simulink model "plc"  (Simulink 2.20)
settings: Solver=ode45  StartTime=0.0  StopTime=1000  RelTol=1e-3  AbsTol=1e-6
undefined symbols (not defined in the file or in its folder): Manual

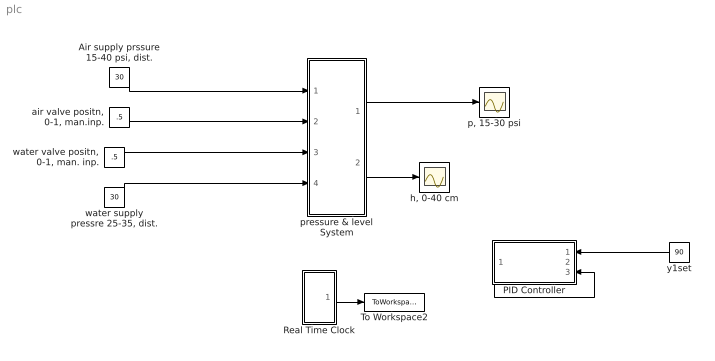
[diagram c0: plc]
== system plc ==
  "Air supply prssure 15-40 psi, dist." : Constant  Value=30
  PID Controller : Subsystem  Orientation=left  mask(Real PID Controller){am_flag=Manual, co=1, Ts=1, Kc=1, taui=10000, taud=0, co_max=100, co_min=0, al=0}
      mask prompts: am_flag "Auto/Manual Switch"; co "Manual Controller Output"; Ts "Sample Time,Ts"; Kc "Kc: Proportional Gain: Negative for DIRECT Action"; taui "taui: Integral time"; taud "Derivative Time, taud"; co_max "Upper limit for controller output"; co_min "Lower limit for controller output"; al "Noise filter tim const, al"
      mask help: Programmed by Babu Joseph, Washington Universtiy in St. Louis, 1998
  Real Time Clock : Subsystem  mask(Sample time){Ts=1}
      mask prompts: Ts "Sample time"
      mask help: This block is used to set the sample time.
  To Workspace2 : ToWorkspace  VariableName=t  SampleTime=1
  "air valve positn, 0-1, man.inp." : Constant  Value=.5
  "h, 0-40 cm" : Scope
  "p, 15-30 psi" : Scope
  pressure & level System : Subsystem  mask{A=100, hinit=20, pinit=25, Ts=1}
      mask prompts: A "area"
  "water supply pressre 25-35, dist." : Constant  Value=30
  "water valve positn, 0-1, man. inp." : Constant  Value=.5
  y1set : Constant  Orientation=left  Value=90
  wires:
  "Air supply prssure 15-40 psi, dist."/1 -> pressure & level System/1(In1)
  pressure & level System/1(p) -> "p, 15-30 psi"/1
  "air valve positn, 0-1, man.inp."/1 -> pressure & level System/2(In2)
  y1set/1 -> PID Controller/1(setpt)
  ? -> PID Controller/2(meas)
  PID Controller/1(output) -> PID Controller/3(out_fdbk)
  Real Time Clock/1("Clock ") -> To Workspace2/1
  "water valve positn, 0-1, man. inp."/1 -> pressure & level System/3(xw)
  "water supply pressre 25-35, dist."/1 -> pressure & level System/4(pw)
  pressure & level System/2(h) -> "h, 0-40 cm"/1

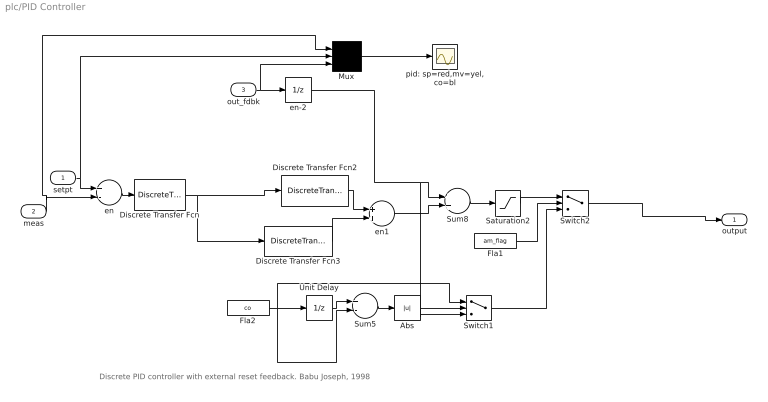
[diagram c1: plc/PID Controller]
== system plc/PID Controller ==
  note: Discrete PID controller with external reset feedback. Babu Joseph, 1998
  setpt : Inport  Port=1  PortWidth=-1  SampleTime=-1
  meas : Inport  Port=2  PortWidth=-1  SampleTime=-1
  out_fdbk : Inport  Port=3  PortWidth=-1  SampleTime=-1
  Abs : Abs
  Discrete Transfer Fcn : DiscreteTransferFcn  Numerator="[Ts   0]"  Denominator="[(al+Ts)  -al]"  SampleTime=Ts
  Discrete Transfer Fcn2 : DiscreteTransferFcn  Numerator="Kc*[ (1+Ts/taui)  -1 ]"  Denominator="[ 1  0 ]"  SampleTime=Ts
  Discrete Transfer Fcn3 : DiscreteTransferFcn  Numerator=Kc*taud*[1 -2 1]  Denominator=[ 1 0 0]  SampleTime=Ts
  Fla1 : Constant  Value=am_flag
  Fla2 : Constant  Value=co
  Mux : Mux  Inputs=3
  Saturation2 : Saturate  UpperLimit=co_max  LowerLimit=co_min
  Sum5 : Sum  Inputs=+-
  Sum8 : Sum  Inputs=++
  Switch1 : Switch  Threshold=0.0001
  Switch2 : Switch  Threshold=1.5
  Unit Delay : UnitDelay  X0=0  SampleTime=Ts
  en : Sum  Inputs=+-
  en-2 : UnitDelay  X0=co  SampleTime=Ts
  en1 : Sum  Inputs=++
  pid: sp=red,mv=yel,co=bl : Scope
  output : Outport  Port=1  InitialOutput=0
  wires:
  Discrete Transfer Fcn/1 -> Discrete Transfer Fcn3/1, Discrete Transfer Fcn2/1
  en/1 -> Discrete Transfer Fcn/1
  setpt/1 -> Mux/2, en/1
  en1/1 -> Sum8/2
  Discrete Transfer Fcn2/1 -> en1/1
  Discrete Transfer Fcn3/1 -> en1/2
  Switch2/1 -> output/1
  en-2/1 -> Switch1/3, Sum8/1
  Switch1/1 -> Switch2/3
  Unit Delay/1 -> Sum5/1
  Fla2/1 -> Unit Delay/1, Sum5/2, Switch1/1
  Sum5/1 -> Abs/1
  Abs/1 -> Switch1/2
  Fla1/1 -> Switch2/2
  Saturation2/1 -> Switch2/1
  Sum8/1 -> Saturation2/1
  meas/1 -> en/2, Mux/1
  out_fdbk/1 -> en-2/1, Mux/3
  Mux/1 -> pid: sp=red,mv=yel,co=bl/1

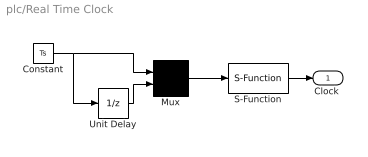
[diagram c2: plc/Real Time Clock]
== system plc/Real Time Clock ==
  Constant : Constant  Value=Ts
  Mux : Mux  Inputs=2
  S-Function : S-Function  FunctionName=wait3  PortCounts=[]  SFunctionModules=''
  Unit Delay : UnitDelay  X0=0  SampleTime=Ts
  "Clock " : Outport  Port=1  InitialOutput=0
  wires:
  S-Function/1 -> "Clock "/1
  Mux/1 -> S-Function/1
  Unit Delay/1 -> Mux/2
  Constant/1 -> Mux/1, Unit Delay/1

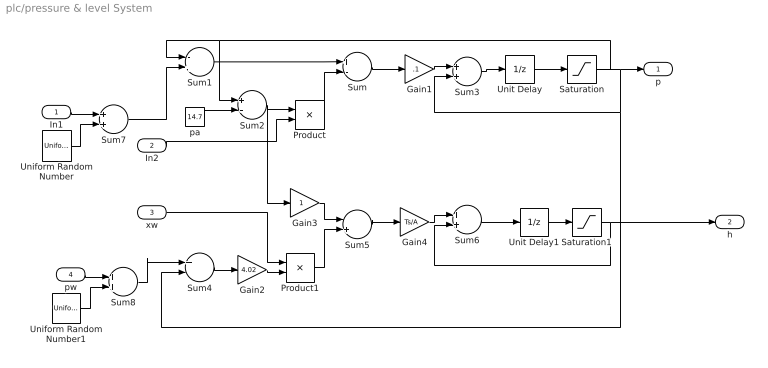
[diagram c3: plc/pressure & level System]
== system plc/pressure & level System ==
  In1 : Inport  Port=1  PortWidth=-1  SampleTime=-1
  In2 : Inport  Port=2  PortWidth=-1  SampleTime=-1
  xw : Inport  Port=3  PortWidth=-1  SampleTime=-1
  pw : Inport  Port=4  PortWidth=-1  SampleTime=-1
  Gain1 : Gain  Gain=.1
  Gain2 : Gain  Gain=4.02
  Gain3 : Gain  Gain=1
  Gain4 : Gain  Gain=Ts/A
  Product : Product  Inputs=2
  Product1 : Product  Inputs=2
  Saturation : Saturate  UpperLimit=30  LowerLimit=14.7
  Saturation1 : Saturate  UpperLimit=40  LowerLimit=1
  Sum : Sum  Inputs=+-
  Sum1 : Sum  Inputs=-+
  Sum2 : Sum  Inputs=+-
  Sum{3,6..8} (4 alike) : Sum  Inputs=++
  Sum4 : Sum  Inputs=+-
  Sum5 : Sum  Inputs=-+
  Uniform Random Number : UniformRandomNumber  Minimum=-1  Maximum=1  Seed=0  SampleTime=1
  Uniform Random Number1 : UniformRandomNumber  Minimum=-2  Maximum=2  Seed=0  SampleTime=1
  Unit Delay : UnitDelay  X0=pinit  SampleTime=Ts
  Unit Delay1 : UnitDelay  X0=hinit  SampleTime=Ts
  pa : Constant  Value=14.7
  p : Outport  Port=1  InitialOutput=0
  h : Outport  Port=2  InitialOutput=0
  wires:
  pa/1 -> Sum2/2
  Sum1/1 -> Sum/1
  Saturation/1 -> Sum1/1, Sum2/1, p/1, Sum3/2, Sum4/2
  Unit Delay/1 -> Saturation/1
  Sum/1 -> Gain1/1
  Gain1/1 -> Sum3/1
  Sum3/1 -> Unit Delay/1
  Product/1 -> Sum/2
  In2/1 -> Product/2
  Sum4/1 -> Gain2/1
  Gain2/1 -> Product1/2
  xw/1 -> Product1/1
  Sum2/1 -> Product/1, Gain3/1
  Gain3/1 -> Sum5/1
  Product1/1 -> Sum5/2
  Sum5/1 -> Gain4/1
  Sum6/1 -> Unit Delay1/1
  Unit Delay1/1 -> Saturation1/1
  Gain4/1 -> Sum6/1
  Saturation1/1 -> h/1, Sum6/2
  In1/1 -> Sum7/1
  Uniform Random Number/1 -> Sum7/2
  Sum7/1 -> Sum1/2
  pw/1 -> Sum8/1
  Uniform Random Number1/1 -> Sum8/2
  Sum8/1 -> Sum4/1
